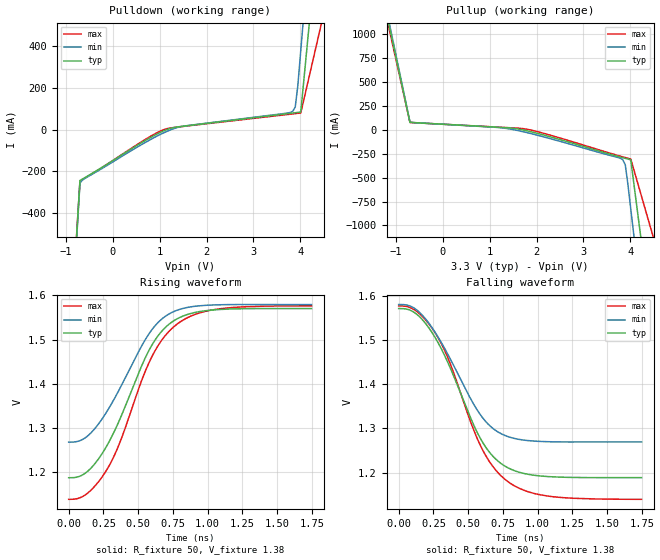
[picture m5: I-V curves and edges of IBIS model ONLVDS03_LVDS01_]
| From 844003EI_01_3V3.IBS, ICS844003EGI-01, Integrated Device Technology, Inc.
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[Model]   ONLVDS03_LVDS01_
Model_type   Output
Polarity   Non-Inverting
|   typ   min   max
C_comp   2pF   1.5pF   2.5pF
Vmeas = 1.38V
Rref = 50
Cref = 0
Vref = 1.38V
|   typ   min   max
[Voltage range]   3.3V   3.135V   3.465V
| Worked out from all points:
|   slope of the pulldown table from 0 to 0.495 V, typ, clamps not added: 7.07 ohm
|   slope of the pullup table from 0 to 0.495 V, typ, clamps not added: 37.1 ohm
|   rising waveform, R_fixture 50, V_fixture 1.38: 20-80 % time 328ps typ, 325ps min, 338ps max; typ from 1.19 V to 1.57 V
|   falling waveform, R_fixture 50, V_fixture 1.38: 20-80 % time 328ps typ, 325ps min, 338ps max; typ from 1.57 V to 1.19 V
[Pulldown]
|Voltage   I (typ)   I (min)   I (max)
-3.3V     -12.71A    -11.01A    -15.57A
-1.22V    -2.163A    -2.22A     -2.109A
-700mV    -243.4mA   -255.4mA   -245.9mA
-591mV    -228.8mA   -232.9mA   -231.1mA
975.4mV   -17.01mA   -26.96mA   -10.67mA
1.461V    15.81mA    15.12mA    14.81mA
3.838V    79.94mA    87.99mA    75.84mA
3.892V    81.43mA    109mA      77.23mA
3.946V    83mA       208.7mA    78.62mA
4.01V     85.14mA    379.8mA    80.26mA
4.528V    1.294A     1.77A      585mA
6.6V      7.984A     7.36A      9.101A
[Pullup]
|Voltage   I (typ)   I (min)   I (max)
-3.3V     7.976A     6.908A     9.771A
-1.22V    1.261A     1.299A     1.219A
-700mV    77.14mA    81.32mA    75.55mA
1.191V    25.7mA     22.95mA    26.95mA
1.732V    -4.365mA   -22.72mA   10.36mA
3.784V    -284.8mA   -297.7mA   -275.6mA
3.838V    -291.9mA   -312.5mA   -283.1mA
3.892V    -299mA     -365.2mA   -290.5mA
3.946V    -306.1mA   -559.4mA   -297.8mA
4.01V     -314.8mA   -828mA     -306.5mA
4.528V    -2.273A    -3.003A    -1.186A
6.6V      -12.73A    -11.74A    -14.49A
[Ramp]
|   typ   min   max
dV/dt_r   0.305/0.507n   0.248/0.487n   0.349/0.546n
dV/dt_f   0.305/0.507n   0.248/0.487n   0.349/0.546n
R_load =   50.0000
[Rising Waveform]
R_fixture = 50
V_fixture = 1.38   |Vcc_typ
V_fixture_min = 1.38 |Vcc_min
V_fixture_max = 1.38 |Vcc_max
C_fixture = 0.0p
| Time   typ   min   max
0s        1.188V     1.268V     1.139V
131.4ps   1.201V     1.281V     1.152V
271.5ps   1.258V     1.336V     1.204V
366.1ps   1.318V     1.388V     1.266V
588.6ps   1.482V     1.518V     1.455V
676.2ps   1.521V     1.548V     1.501V
772.5ps   1.545V     1.565V     1.533V
903.9ps   1.561V     1.575V     1.556V
1.074ns   1.568V     1.578V     1.569V
1.748ns   1.57V      1.579V     1.576V
[Falling Waveform]
R_fixture = 50
V_fixture = 1.38   |Vcc_typ
V_fixture_min = 1.38 |Vcc_min
V_fixture_max = 1.38 |Vcc_max
C_fixture = 0.0p
| Time   typ   min   max
0s        1.571V     1.58V      1.576V
131.4ps   1.557V     1.567V     1.564V
271.5ps   1.5V       1.512V     1.511V
366.1ps   1.44V      1.46V      1.45V
588.6ps   1.277V     1.33V      1.261V
676.2ps   1.238V     1.3V       1.214V
772.5ps   1.213V     1.283V     1.183V
903.9ps   1.198V     1.273V     1.16V
1.074ns   1.191V     1.27V      1.147V
1.748ns   1.189V     1.269V     1.139V
